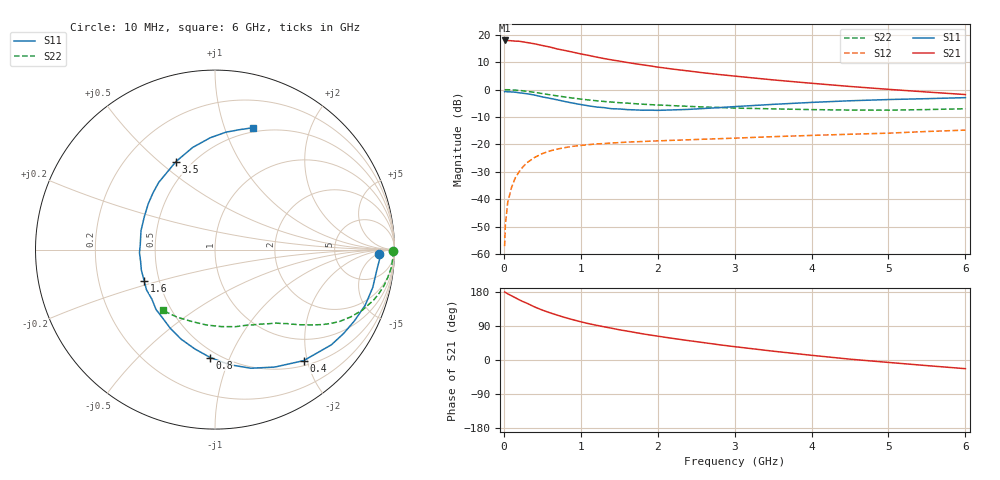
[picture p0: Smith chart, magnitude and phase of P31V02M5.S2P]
! SIEMENS Small Signal Semiconductors
! BFP181
! Si NPN RF Bipolar Junction Transistor in SOT143
! VCE = 1 V  IC = 2.5 mA
! Common Emitter S-Parameters:  March  1996
# GHz  S  MA  R  50
!  f  S11  S21  S12  S22
! GHz  MAG  ANG  MAG  ANG  MAG  ANG  MAG  ANG
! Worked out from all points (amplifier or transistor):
!   36 points, 10 MHz to 6 GHz, reference 50 ohm
!   highest |S21| = 17.9 dB at 10 MHz (marker M1)
!   |S21| within 3 dB of that: start of sweep to 681.5 MHz
!   unconditionally stable (mu >= 1): 2.06 GHz to end of sweep
!   at 250 MHz: K = 0.15, MSG = 22.7 dB, |S12| = -28.1 dB
!   at 1.4 GHz: K = 0.76, MSG = 15.1 dB, |S12| = -19.5 dB
!   at 6 GHz: K = 1.18, MAG = 3.9 dB, |S12| = -14.8 dB
!   S11 on the Smith chart (normalised r, x): 10 MHz: 20, -6; 400 MHz: 0.58, -1.94; 800 MHz: 0.45, -0.85; 1.6 GHz: 0.41, -0.17; 3.5 GHz: 0.41, +0.57; 6 GHz: 0.46, +1.26
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0.01  0.9118 -1.5  7.834 179.2  0.0014 83.0  0.9943 -0.5
0.02  0.9206 -2.8  7.821 178.5  0.0034 88.6  0.9917 -1.2
0.05  0.9095 -6.7  7.813 174.7  0.0087 88.4  0.9915 -3.1
0.1  0.9039 -13.5  7.727 169.5  0.0164 81.5  0.986 -6.2
0.2  0.8724 -27.1  7.575 158.9  0.032 74.7  0.9625 -12.1
0.25  0.8556 -33.1  7.381 154.0  0.0393 70.7  0.9456 -15.0
0.4  0.7916 -51.4  6.807 140.0  0.0579 60.8  0.8881 -22.3
0.5  0.7344 -63.0  6.343 131.7  0.068 54.7  0.8438 -26.4
0.6  0.6904 -73.2  5.938 124.5  0.0761 50.2  0.8023 -29.9
0.7  0.6463 -82.8  5.461 118.0  0.0825 46.5  0.764 -32.6
0.8  0.602 -92.5  5.126 111.8  0.0878 42.7  0.7301 -34.9
1  0.5333 -110.8  4.451 100.9  0.0957 37.1  0.6697 -38.8
1.1  0.5046 -119.5  4.193 96.0  0.099 34.9  0.6461 -40.4
1.3  0.4682 -134.6  3.674 87.7  0.1037 31.2  0.6066 -43.3
1.6  0.4311 -156.4  3.116 76.4  0.1101 27.5  0.5651 -46.8
1.9  0.4212 -177.6  2.696 66.0  0.1145 25.0  0.5307 -50.5
2.2  0.4256 165.6  2.352 56.9  0.1188 23.1  0.5083 -54.4
2.8  0.4685 137.4  1.876 40.2  0.1271 20.4  0.4707 -63.0
3.5  0.5366 113.9  1.498 23.3  0.1384 17.7  0.4444 -75.1
4.5  0.6239 92.4  1.137 2.2  0.1532 13.3  0.4227 -96.5
5.5  0.6817 78.5  0.901 -14.8  0.172 10.0  0.4313 -119.1
6  0.7118 72.6  0.81 -22.9  0.1823 7.6  0.4467 -130.6
